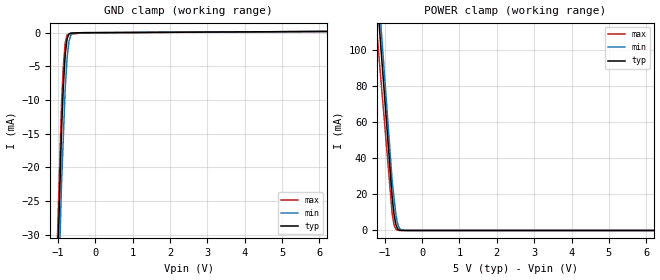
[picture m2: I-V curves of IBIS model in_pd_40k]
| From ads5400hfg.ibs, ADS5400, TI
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[Model] in_pd_40k
Model_type Input
Vinl = 800.000mV
Vinh = 2.00000V
C_comp 250.000fF 232.000fF 272.000fF
| variable typ   min   max
[Voltage Range] 5.00000V 4.75000V 5.25000V
[POWER Clamp Reference] 5.00000V 4.75000V 5.25000V
[GND Clamp Reference] 0.00000V 0.00000V 0.00000V
[Temperature Range] 25   85   -40
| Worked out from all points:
|   GND clamp passes 1 mA (typ) near -0.75 V on its own axis
|   POWER clamp passes 1 mA (typ) near -0.65 V on its own axis
[GND Clamp]
-5V       -794.6mA   -841.4mA   -752.9mA
-900mV    -14.73mA   -22.62mA   -10.85mA
-850mV    -7.878mA   -15.44mA   -4.891mA
-800mV    -3.227mA   -8.256mA   -1.501mA
-750mV    -893.9uA   -3.756mA   -307uA
-700mV    -197.2uA   -1.289mA   -274.2uA
-650mV    -60.98uA   -393uA     -241.3uA
-600mV    -53.76uA   -103.9uA   -208.4uA
-375mV    -21.25uA   -38.04uA   -60.42uA
-325mV    -14.02uA   -23.4uA    -58.63uA
-300mV    -13.32uA   -16.09uA   -57.73uA
10V       276.8uA    277.9uA    311uA
[POWER Clamp]
-5V       1.175A     1.232A     1.048A
-1.05V    87.76mA    99.58mA    71.45mA
-800mV    18.93mA    27.93mA    9.612mA
-750mV    9.168mA    18.42mA    3.199mA
-700mV    3.277mA    8.919mA    652.3uA
-650mV    784.4uA    3.506mA    126.3uA
-600mV    145.4uA    1.029mA    22.9uA
-550mV    29.66uA    236.8uA    20.21uA
-400mV    13.48uA    10.72uA    12.12uA
10V       0A         0A         0A
